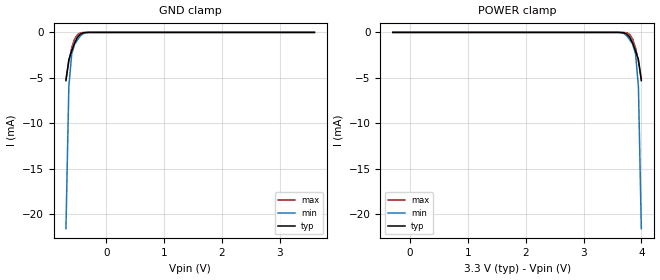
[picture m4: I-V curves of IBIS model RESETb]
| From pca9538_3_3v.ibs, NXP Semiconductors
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[Model]   RESETb
Model_type Input
Vinh=2.31
Vinl=0.99
C_comp   1.73p   1.7p   1.78p
[Temperature Range] 27   85   -40
[Voltage Range]   3.3   3   3.6
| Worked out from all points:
|   GND clamp passes 1 mA (typ) near -0.54 V on its own axis
[GND Clamp]
-700mV    -5.302mA   -21.58mA   -5.122mA
-650mV    -2.995mA   -5.963mA   -3.206mA
-600mV    -2.04mA    -2.358mA   -1.687mA
-550mV    -1.169mA   -1.297mA   -720.1uA
-500mV    -525.2uA   -816.9uA   -228.9uA
-450mV    -185.2uA   -388.2uA   -49.68uA
-400mV    -48.21uA   -135uA     -7.763uA
-250mV    -208.1nA   -1.277uA   -8.827nA
3.6V      65.11pA    250.9pA    47.06pA
[POWER Clamp]
-300mV    65.11pA    250.9pA    47.06pA
3.55V     -208nA     -1.277uA   -8.827nA
3.7V      -48.21uA   -135uA     -7.763uA
3.75V     -185.2uA   -388.2uA   -49.68uA
3.8V      -525.2uA   -816.9uA   -228.9uA
3.85V     -1.169mA   -1.297mA   -720.1uA
3.9V      -2.04mA    -2.358mA   -1.687mA
3.95V     -2.995mA   -5.963mA   -3.206mA
4V        -5.302mA   -21.58mA   -5.122mA
